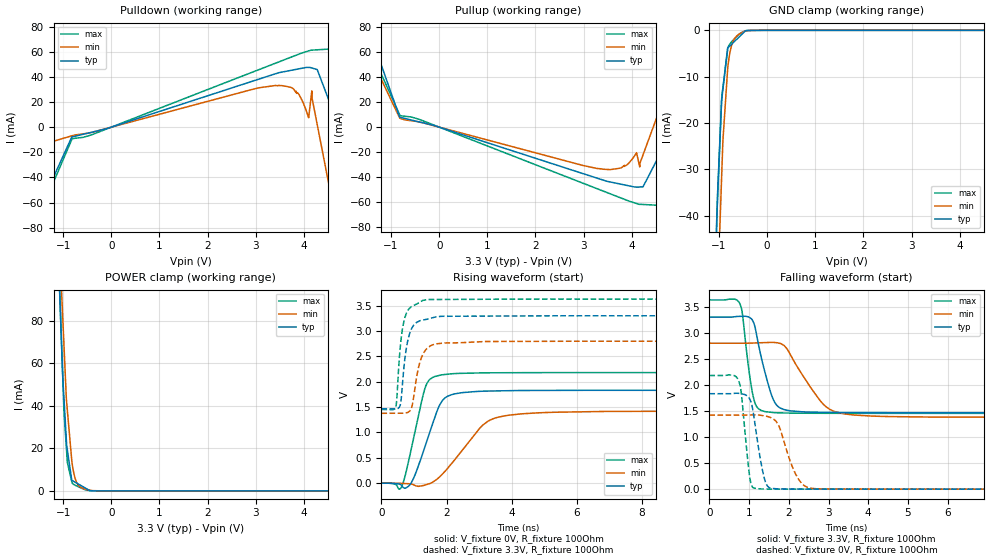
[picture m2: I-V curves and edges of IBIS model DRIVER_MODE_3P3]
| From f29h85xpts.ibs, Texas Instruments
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|   Model Cell DRIVER_MODE_3P3
|DRIVER_MODE_3P3
[Model]   DRIVER_MODE_3P3
Model_type   I/O
Polarity   Non-Inverting
Enable   Active-Low
Vinl = 0.8
Vinh = 2
Vmeas = 1.65
Vref = 0
Cref = 15pF
Rref = 100M
|   typ   min   max
C_comp   0.36pF   0.33pF   0.386pF
[Model Spec]
Vinl   0.8   0.8   0.8
Vinh   2   2   2
[Temperature Range]   25   155   -40
[Voltage Range]   3.3   2.8   3.63
| Nom Voltages:
|   BIASFET=3.3, VDD=1.23, VDDS=3.3, VSS=0
| Min Voltages:
|   BIASFET=2.97, VDD=1.08, VDDS=2.8, VSS=0
| Max Voltages:
|   BIASFET=3.63, VDD=1.32, VDDS=3.63, VSS=0
[Pullup Reference]   3.3   2.8   3.63
[Pulldown Reference]   0   0   0
[Power Clamp Reference]   3.3   2.8   3.63
[GND Clamp Reference]   0   0   0
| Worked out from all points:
|   slope of the pulldown table from 0 to 0.495 V, typ, clamps not added: 80 ohm
|   slope of the pullup table from 0 to 0.495 V, typ, clamps not added: 80.1 ohm
|   GND clamp passes 1 mA (typ) near -0.54 V on its own axis
|   POWER clamp passes 1 mA (typ) near -0.51 V on its own axis
|   falling waveform, V_fixture 3.3V, R_fixture 100Ohm: 20-80 % time 357ps typ, 743ps min, 216ps max; typ from 3.3 V to 1.47 V
|   rising waveform, V_fixture 0V, R_fixture 100Ohm: 20-80 % time 587ps typ, 1.08ns min, 449ps max; typ from 0 V to 1.83 V
|   rising waveform, V_fixture 3.3V, R_fixture 100Ohm: 20-80 % time 228ps typ, 275ps min, 198ps max; typ from 1.47 V to 3.3 V
|   falling waveform, V_fixture 0V, R_fixture 100Ohm: 20-80 % time 230ps typ, 385ps min, 166ps max; typ from 1.83 V to 0 V
[Pulldown]
|   Voltage   I(typ)   I(min)   I(max)
-3.3V     -9.485mA   -5.677mA   -12.22mA
-3.215V   -59.69mA   -44.77mA   -94.86mA
-1.569V   -70.41mA   -54.46mA   -76.72mA
-813.8mV  -7.792mA   -6.822mA   -9.249mA
4.166V    47.12mA    28.81mA    61.3mA
4.592V    14.16mA    -59.79mA   57.49mA
6.077V    -22.02mA   -68.82mA   -17.35mA
6.176V    -21.01mA   9.017mA    -22.34mA
6.518V    -17.53mA   -77.48mA   11.63mA
6.52V     -17.5mA    9.407mA    11.89mA
6.544V    570.1mA    856.6mA    14.39mA
6.6V      1.983A     2.894A     1.856A
[GND Clamp]
|   Voltage   I(typ)   I(min)   I(max)
-3.3V     -1.461A    -1.198A    -2.144A
-1.049V   -42.6mA    -64.96mA   -41.2mA
-1.03V    -35.53mA   -57.63mA   -36.62mA
-1.02V    -32.95mA   -53.79mA   -33.93mA
-946.8mV  -15.29mA   -32.13mA   -15.46mA
-942.3mV  -14.88mA   -30.8mA    -14.33mA
-918.7mV  -12.73mA   -23.81mA   -12.37mA
-821.3mV  -3.843mA   -8.552mA   -4.277mA
-789.8mV  -3.526mA   -5.836mA   -3.211mA
-681.3mV  -2.434mA   -1.871mA   -1.849mA
-446.7mV  -75.06uA   -176uA     -115.4uA
6.6V      0A         0A         0A
[Pullup]
|   Voltage   I(typ)   I(min)   I(max)
-3.3V     10.42mA    7.234mA    13.28mA
-3.215V   75.69mA    81.16mA    91.4mA
-1.562V   88.99mA    96.89mA    72.97mA
-1.382V   69.23mA    19.25mA    57.61mA
3.274V    -40.75mA   -33.04mA   -49.17mA
4.602V    -20.34mA   15.39mA    -62.62mA
6.077V    5.77mA     22.25mA    21.42mA
6.192V    4.916mA    -17.46mA   27.96mA
6.518V    2.496mA    27.52mA    -8.783mA
6.52V     2.478mA    -19.2mA    -9.054mA
6.544V    -441.8mA   -474.9mA   -11.7mA
6.6V      -1.511A    -1.571A    -1.89A
[POWER Clamp]
|   Voltage   I(typ)   I(min)   I(max)
-3.3V     1.933A     2.239A     2.093A
-1.075V   94.97mA    124.6mA    96.59mA
-1.03V    66.74mA    92.35mA    67.32mA
-1.006V   52.5mA     80.08mA    51.82mA
-980.4mV  42.48mA    67.22mA    36.38mA
-932.9mV  23.7mA     43.1mA     20.22mA
-912.8mV  19.24mA    37.92mA    13.36mA
-821.3mV  5.004mA    14.38mA    4.428mA
-779.3mV  4.459mA    8.484mA    3.039mA
-693.7mV  3.351mA    2.906mA    2.058mA
-583mV    1.918mA    1.147mA    912.8uA
6.6V      0A         0A         0A
[Ramp]
R_load = 100
|   typ   min   max
dV/dt_r   1.09894/5.8601e-10   0.852932/1.07931e-09   1.30833/4.48799e-10
dV/dt_f   1.09983/3.57041e-10   0.853154/7.46023e-10   1.30537/2.16335e-10
[Falling Waveform]
V_fixture = 3.3V
V_fixture_min = 2.8V
V_fixture_max = 3.63V
R_fixture = 100Ohm
C_fixture = 0F
|   Time   V(typ)   V(min)   V(max)
0s        3.3V       2.8V       3.63V
773ps     3.315V     2.8V       3.551V
828.8ps   3.316V     2.8V       3.382V
1.078ns   3.251V     2.803V     1.878V
1.234ns   2.786V     2.807V     1.545V
1.628ns   1.691V     2.815V     1.468V
1.959ns   1.513V     2.69V      1.461V
2.936ns   1.473V     1.582V     1.456V
4.104ns   1.469V     1.402V     1.455V
50ns      1.467V     1.378V     1.454V
[Rising Waveform]
V_fixture = 0V
V_fixture_min = 0V
V_fixture_max = 0V
R_fixture = 100Ohm
C_fixture = 0F
|   Time   V(typ)   V(min)   V(max)
0s        76.6nV     323.4nV    64.42nV
570.7ps   -21.72mV   -1.49mV    -113.4mV
887ps     -19.48mV   -13.93mV   589.6mV
1.262ns   576.2mV    -48.43mV   1.69V
1.405ns   850mV      -23.36mV   1.976V
1.786ns   1.54V      124.5mV    2.126V
2.183ns   1.75V      408.6mV    2.158V
3.269ns   1.816V     1.221V     2.177V
5.056ns   1.829V     1.393V     2.18V
50ns      1.832V     1.422V     2.181V
[Rising Waveform]
V_fixture = 3.3V
V_fixture_min = 2.8V
V_fixture_max = 3.63V
R_fixture = 100Ohm
C_fixture = 0F
|   Time   V(typ)   V(min)   V(max)
0s        1.467V     1.378V     1.454V
440.7ps   1.465V     1.379V     1.502V
561.1ps   1.51V      1.38V      2.556V
623.1ps   1.773V     1.38V      2.941V
754.3ps   2.616V     1.387V     3.327V
874.7ps   2.964V     1.424V     3.455V
1.188ns   3.203V     2.399V     3.572V
1.405ns   3.233V     2.659V     3.619V
3.192ns   3.294V     2.793V     3.626V
50ns      3.3V       2.8V       3.63V
[Falling Waveform]
|Gnd
V_fixture = 0V
V_fixture_min = 0V
V_fixture_max = 0V
R_fixture = 100Ohm
C_fixture = 0F
|   Time   V(typ)   V(min)   V(max)
0s        1.832V     1.422V     2.181V
720.5ps   1.839V     1.421V     2.11V
805ps     1.83V      1.421V     1.836V
1.036ns   1.697V     1.423V     146.2mV
1.262ns   677.2mV    1.421V     5.579mV
1.498ns   33.74mV    1.386V     2.639mV
1.756ns   4.96mV     1.206V     1.179mV
2.248ns   1.89mV     186.4mV    828.5uV
2.709ns   1.092mV    7.953mV    522.9uV
50ns      58.05nV    240.7nV    40.61nV
